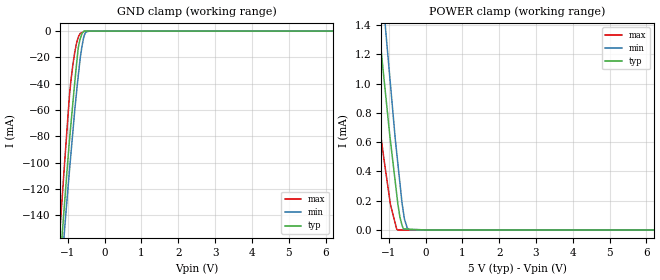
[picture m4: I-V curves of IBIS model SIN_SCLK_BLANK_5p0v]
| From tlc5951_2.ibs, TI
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|   sin_sclk_blank_5p0v Model
[Model]   SIN_SCLK_BLANK_5p0v
Model_type   Input
Vinl = 1.5
Vinh = 3.5
|   typ   min   max
|   (nom PVT)   (Fast PVT)   (slow PVT)
|Average
C_comp   1.178e-12   1.163e-12   1.277e-12
| Where nom  PVT is Nominal Process,  5V,  65C
|   Fast PVT is Strong Process,   5.5V,  -40C
|   Slow PVT is Weak Process,   4.5V,  125C
[Model Spec]
Vinl   1.5   1.35   1.65
Vinh   3.5   3.15   3.85
[Voltage Range]   5   4.5   5.5
|Ambient Temperature   25   85   -40
|Junction Temperature
[Temperature Range]   65   125   -40
[Power Clamp Reference]   5   4.5   5.5
[GND Clamp Reference]   0   0   0
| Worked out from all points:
|   GND clamp passes 1 mA (typ) near -0.59 V on its own axis
|   POWER clamp passes 1 mA (typ) near -1.11 V on its own axis
[GND Clamp]
|   Voltage   I(typ)   I(min)   I(max)
-5V       -1.792A    -1.69A     -1.896A
-1.23V    -183.1mA   -200.9mA   -158.3mA
-1.21V    -175.7mA   -193.9mA   -150mA
-1.153V   -154.3mA   -173.2mA   -126.5mA
-1.084V   -129.1mA   -149.5mA   -98.85mA
-952mV    -82.24mA   -105mA     -47.9mA
-864mV    -54.97mA   -76.92mA   -25.97mA
-720mV    -13.52mA   -34.91mA   -5.134mA
-657.5mV  -5.392mA   -19.32mA   -1.761mA
-563mV    -33.03uA   -4.24mA    -456.5uA
-419mV    0A         0A         0A
10V       0A         0A         0A
[POWER Clamp]
|   Voltage   I(typ)   I(min)   I(max)
-5V       7.099mA    5.5mA      10.13mA
-1.675V   2.51mA     3.175mA    1.555mA
-1.425V   1.809mA    2.407mA    1.049mA
-1.315V   1.515mA    2.069mA    835.1uA
-1.139V   1.062mA    1.529mA    504.1uA
-952mV    608.8uA    994.7uA    173.9uA
-755mV    186.8uA    463.6uA    0A
-695mV    87.28uA    320.8uA    0A
-572mV    7.106uA    74.32uA    0A
-495.5mV  6.147uA    13.38uA    0A
-414.5mV  5.132uA    0A         0A
10V       0A         0A         0A
